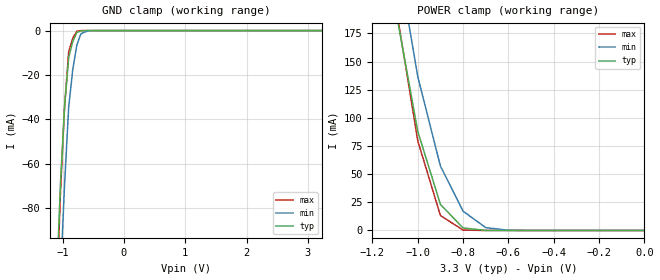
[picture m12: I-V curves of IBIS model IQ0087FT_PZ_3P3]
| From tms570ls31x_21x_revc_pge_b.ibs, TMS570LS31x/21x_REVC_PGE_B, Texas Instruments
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|   Model Cell IQ0087FT_PZ_3P3
|IQ0087FT_PZ_3P3
[Model]   IQ0087FT_PZ_3P3
Model_type   Input
Polarity   Non-Inverting
Vinl =  1.15
Vinh =  1.55
C_comp   1.2p   1.2p   1.2p
[Model Spec]
Vinl   1.15   1.02   1.28
Vinh   1.55   1.45   1.65
[Temperature Range]   25   155   -40
[Voltage Range]   3.3   2.97   3.63
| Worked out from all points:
|   GND clamp passes 1 mA (typ) near -0.77 V on its own axis
|   POWER clamp passes 1 mA (typ) near -0.74 V on its own axis
[POWER_clamp]
|   voltage   I(typ)   I(min)   I(max)
-3.3V     3.541A     4.385A     3.783A
-1.1V     198.7mA    255.1mA    203.4mA
-1.067V   161.8mA    215.6mA    162.1mA
-1.033V   124.9mA    176.1mA    120.8mA
-1V       87.93mA    136.6mA    79.54mA
-900mV    23.11mA    57.15mA    13.26mA
-800mV    2.235mA    17.1mA     350.6uA
-700mV    70.13uA    2.515mA    5.198uA
-600mV    2.318uA    221.3uA    475.8nA
0V        280.4pA    424.1pA    308.7pA
[GND_clamp]
|   voltage   I(typ)   I(min)   I(max)
-3.3V     -2.707A    -2.59A     -3.853A
-1.1V     -116mA     -158.3mA   -124.9mA
-1.033V   -68.83mA   -110.6mA   -72.79mA
-966.7mV  -34.24mA   -69.38mA   -34.32mA
-900mV    -12.23mA   -34.62mA   -9.549mA
-833.3mV  -4.922mA   -17.55mA   -3.434mA
-766.7mV  -866.2uA   -6.476mA   -254.5uA
-700mV    -56.97uA   -1.408mA   -9.482uA
-566.7mV  -2.104uA   -110.8uA   -997.2nA
3.233V    270.2pA    105.1nA    247.6pA
